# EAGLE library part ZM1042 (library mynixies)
Indicator Tube (numeral height 30mm, no filter, side view, long-life typ)
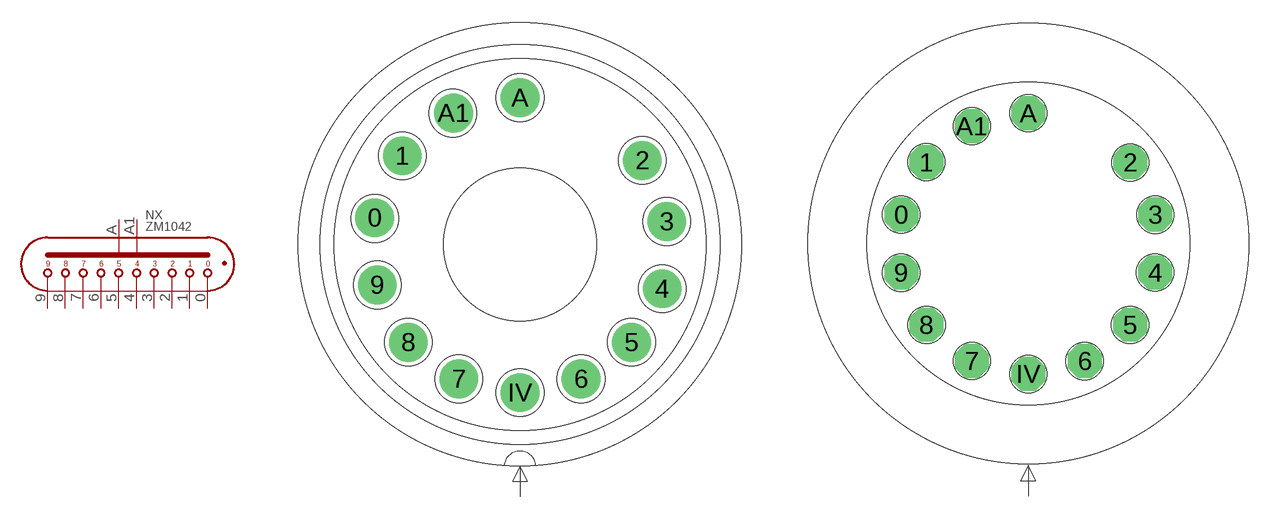
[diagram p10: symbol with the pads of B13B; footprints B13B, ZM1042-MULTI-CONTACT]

Designator prefix NX

## ZM1042-B13B  [B13B]
0  0  pas
1  1  pas
2  2  pas
3  3  pas
4  4  pas
5  5  pas
6  6  pas
7  7  pas
8  8  pas
9  9  pas
A  A1  pas
A1  A2  pas

## ZM1042-B1-B_41.0002  [ZM1042-MULTI-CONTACT]
Pads as for B13B

## ZM1042-1-380758-1  [ZM1042-AMP]
Pads as for B13B

## ZM1042D-SUB  [ZM1042-DSUB]
Pads as for B13B

## ZM1042MILLMAX8331  [ZM1042-8331]
Pads as for B13B

## Footprint B13B (pad centres in mm)
Socket B13B print
drill 1.422 pad 2.54: 0 -9.5,1.75; 1 -7.7,5.8; 2 8,5.5; 3 9.6,1.5; 4 9.3,-2.9; 5 7.3,-6.4; 6 4,-8.8; 7 -4,-8.8; 8 -7.3,-6.4; 9 -9.327,-2.646; A 0,9.6; A1 -4.35,8.6; IV 0,-9.7

## Footprint ZM1042-MULTI-CONTACT (pad centres in mm)
Socket with Multi-Contact (Mini-line Discret Socket Contact) Typ B1-B 41.0002
drill 1.1 pad 2.184 octagon: 0 -8.189,1.869; 1 -6.567,5.237; 2 6.567,5.237; 3 8.189,1.869; 4 8.189,-1.869; 5 6.567,-5.237; 6 3.645,-7.568; 7 -3.645,-7.568; 8 -6.567,-5.237; 9 -8.189,-1.869; A 0,8.4; A1 -3.645,7.568; IV 0,-8.4

## Footprint ZM1042-AMP (pad centres in mm)
Socket with AMP-Discret Socket Contact Typ 1-380758-1
drill 2.3 pad 3.2: 0 -8.189,1.869; 1 -6.567,5.237; 2 6.567,5.237; 3 8.189,1.869; 4 8.189,-1.869; 5 6.567,-5.237; 6 3.645,-7.568; 7 -3.645,-7.568; 8 -6.567,-5.237; 9 -8.189,-1.869; A 0,8.4; A1 -3.645,7.568; IV 0,-8.4

## Footprint ZM1042-DSUB (pad centres in mm)
Socket with D-SUB Sockets
drill 1.6: 0 -8.189,1.869; 1 -6.567,5.237; 2 6.567,5.237; 3 8.189,1.869; 4 8.189,-1.869; 5 6.567,-5.237; 6 3.645,-7.568; 7 -3.645,-7.568; 8 -6.567,-5.237; 9 -8.189,-1.869; A 0,8.4; A1 -3.645,7.568; IV 0,-8.4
